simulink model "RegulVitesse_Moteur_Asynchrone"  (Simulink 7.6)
settings: Solver=ode23tb  StartTime=0.0  StopTime=N  MaxStep=1e-4  MinStep=1e-5  RelTol=1e-4  AbsTol=1e-4
InitFcn:
  | clear all
  | close all
  | clc
  | 
  | 
  | N=800;
StopFcn:
  | close all
  | load tensionVab.mat
  | plot(x(1,:),x(2,:))
  | title('Tension entre les phases A et B')
  | xlabel('temps')
  | grid
libraries: powerlib x7, simulink x1

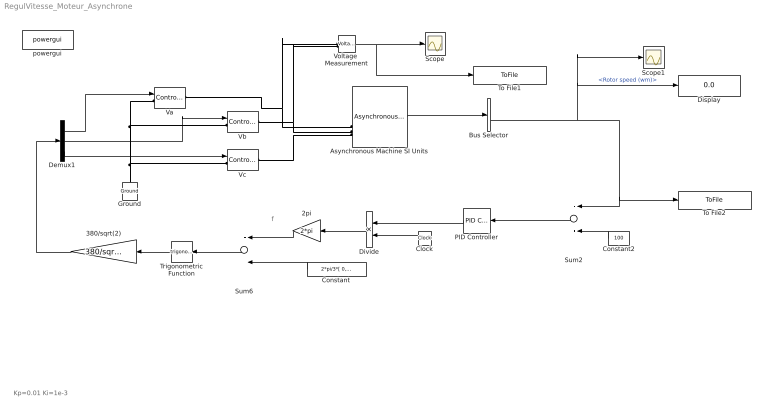
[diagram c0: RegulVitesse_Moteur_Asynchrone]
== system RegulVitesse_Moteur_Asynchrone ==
  note: Kp=0.01 Ki=1e-3
  note: f
  2pi : Gain  Gain=2*pi
  380/sqrt(2) : Gain  Gain=380/sqrt(2)
  Asynchronous Machine SI Units : powerlib/Machines/Asynchronous Machine SI Units  DialogController=POWERSYS.PowerSysDialog  SystemSampleTime=-1  PresetModel=No  MechanicalLoad=Torque Tm  ShowDetailedParameters=on  RotorType=Squirrel-cage  ReferenceFrame=Stationary  NominalParameters=[ 3800, 380, 60 ]  Stator=[ 0.029 0.226/377]  Rotor=[ 0.022 0.226/377]  Cage1=[ 0.022 0.226/377]  Cage2=[ 0.022 0.226/377]  Lm=13.04/377  Mechanical="[ 63.87 0  2 ]"  PolePairs=2  InitialConditions=[1 0 0 0 0 0 0 0]  Units=SI  LoadFlowParameters=1492000  SimulateSaturation=off  Saturation=[14.03593122, 27.81365428, 53.79336849, 72.68890987, 97.98006896, 148.6815601, 215.7428561, 302.9841135, 428.7778367 ; 230, 322, 414, 460, 506, 552, 598, 644, 690]  TsPowergui=0  TsBlock=-1  IterativeModel=Forward Euler
  Bus Selector : BusSelector  OutputSignals=Stator measurements.Stator current is_a (A),Mechanical.Rotor speed (wm)
  Clock : Clock
  Constant : Constant  Value=2*pi/3*[ 0,-1,1 ]
  Constant2 : Constant  Value=100
  Demux1 : Demux  Outputs=3
  Display : Display
  Divide : Product  Inputs=**
  Ground : powerlib/Elements/Ground  DialogController=POWERSYS.PowerSysDialog  PhysicalDomain=powersysdomain  SubClassName=unknown  LeftPortType=p1  RightPortType=p1  LConnTagsString=a
  PID Controller : simulink/Continuous/PID Controller  DialogController=pidpack.PIDConfig.pidDDGCreate  DialogControllerArgs=DataTag0  SystemSampleTime=-1  Controller=PID  TimeDomain=Continuous-time  SampleTime=1  IntegratorMethod=Forward Euler  FilterMethod=Forward Euler  Form=Parallel  P=1e-3  I=0.5e-4  D=0  N=100  InitialConditionSource=internal  InitialConditionForIntegrator=0  InitialConditionForFilter=0  ExternalReset=none  LimitOutput=off  UpperSaturationLimit=inf  LowerSaturationLimit=-inf  LinearizeAsGain=off  AntiWindupMode=none  Kb=1  TrackingMode=off  Kt=1  PParamMin=[]  PParamMax=[]  IParamMin=[]  IParamMax=[]  DParamMin=[]  DParamMax=[]  NParamMin=[]  NParamMax=[]  KbParamMin=[]  KbParamMax=[]  KtParamMin=[]  KtParamMax=[]  POutMin=[]  POutMax=[]  IOutMin=[]  IOutMax=[]  DOutMin=[]  DOutMax=[]  NOutMin=[]  NOutMax=[]  KbOutMin=[]  KbOutMax=[]  KtOutMin=[]  KtOutMax=[]  IntegratorOutMin=[]  IntegratorOutMax=[]  FilterOutMin=[]  FilterOutMax=[]  SumOutMin=[]  SumOutMax=[]  SumI1OutMin=[]  SumI1OutMax=[]  SumI2OutMin=[]  SumI2OutMax=[]  SumI3OutMin=[]  SumI3OutMax=[]  SumDOutMin=[]  SumDOutMax=[]  SaturationOutMin=[]  SaturationOutMax=[]  IntegratorContinuousStateAttributes=''  IntegratorStateMustResolveToSignalObject=off  IntegratorRTWStateStorageClass=Auto  FilterContinuousStateAttributes=''  FilterStateMustResolveToSignalObject=off  FilterRTWStateStorageClass=Auto
  Scope : Scope
  Scope1 : Scope
  Sum2 : Sum  Inputs=-+
  Sum6 : Sum
  To File1 : ToFile  Filename=tensionVab  MatrixName=x
  To File2 : ToFile  Filename=tensionVab  MatrixName=x
  Trigonometric Function : Trigonometry
  Va : powerlib/Electrical Sources/Controlled Voltage Source  Description=source block  DialogController=POWERSYS.PowerSysDialog  SystemSampleTime=-1  Initialize=on  Source_Type=AC  Amplitude=0  Phase=0  Frequency=0  Measurements=None
  Vb : powerlib/Electrical Sources/Controlled Voltage Source  Description=source block  DialogController=POWERSYS.PowerSysDialog  SystemSampleTime=-1  Initialize=on  Source_Type=AC  Amplitude=0  Phase=0  Frequency=0  Measurements=None
  Vc : powerlib/Electrical Sources/Controlled Voltage Source  Description=source block  DialogController=POWERSYS.PowerSysDialog  SystemSampleTime=-1  Initialize=on  Source_Type=AC  Amplitude=0  Phase=0  Frequency=0  Measurements=None
  Voltage  Measurement : powerlib/Measurements/Voltage Measurement  DialogController=POWERSYS.PowerSysDialog  SystemSampleTime=-1  PhasorSimulation=off  OutputType=Complex  PSBequivalent=0
  powergui : powerlib/powergui  Priority=2  SystemSampleTime=-1  SimulationMode=Continuous  SampleTime=1e-5  frequency=60  SPID=off  DisableSnubberDevices=off  DisableRonSwitches=off  DisableVfSwitches=off  SwTol=0  Interpol=off  frequencyindice=60  echomessages=off  HookPort=off  DisplayEquations=off  FunctionMessages=off  EnableUseOfTLC=off  x0status=blocks  RestoreLinks=warning  ResistiveCurrentMeasurement=off  Frange=[0:2:500]  Ylog=off  Xlog=on  ShowGrid=off  save=off  variable=ZData  ZoomFFT=on  StartTime=0.0  cycles=1  DisplayStyle=1  fundamental=60  FreqAxis=off  MaxFrequency=1000  frequencyindicesteady=1  RmsSteady=1  display=off  Ts=0  methode=off
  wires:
  Asynchronous Machine SI Units/1 -> Bus Selector/1
  Bus Selector/2 -> Display/1, Scope1/1, Sum2/1, To File2/1  "<Rotor speed (wm)>"
  2pi/1 -> Sum6/1
  Constant/1 -> Sum6/2
  Trigonometric Function/1 -> 380/sqrt(2)/1
  Demux1/1 -> Va/1
  Demux1/2 -> Vb/1
  Demux1/3 -> Vc/1
  Clock/1 -> Divide/2
  Divide/1 -> 2pi/1
  380/sqrt(2)/1 -> Demux1/1
  Sum6/1 -> Trigonometric Function/1
  Sum2/1 -> PID Controller/1
  Constant2/1 -> Sum2/2
  PID Controller/1 -> Divide/1
  Voltage  Measurement/1 -> Scope/1, To File1/1
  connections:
  Vb/RConn1 -- Asynchronous Machine SI Units/LConn2 -- Voltage  Measurement/LConn2
  Vc/RConn1 -- Asynchronous Machine SI Units/LConn3
  Ground/LConn1 -- Vc/LConn1 -- Va/LConn1 -- Vb/LConn1
  Va/RConn1 -- Asynchronous Machine SI Units/LConn1 -- Voltage  Measurement/LConn1
